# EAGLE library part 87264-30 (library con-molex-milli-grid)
RECEPTACAL
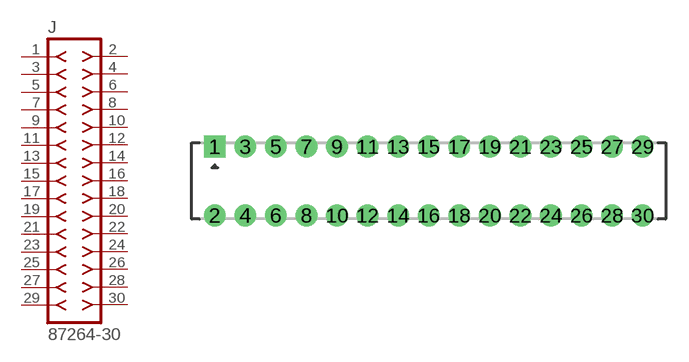
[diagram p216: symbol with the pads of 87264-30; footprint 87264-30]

Designator prefix J

## 87264-30  [87264-30]
1  1  pas
2  2  pas
3  3  pas
4  4  pas
5  5  pas
6  6  pas
7  7  pas
8  8  pas
9  9  pas
10  10  pas
11  11  pas
12  12  pas
13  13  pas
14  14  pas
15  15  pas
16  16  pas
17  17  pas
18  18  pas
19  19  pas
20  20  pas
21  21  pas
22  22  pas
23  23  pas
24  24  pas
25  25  pas
26  26  pas
27  27  pas
28  28  pas
29  29  pas
30  30  pas

## Footprint 87264-30 (pad centres in mm)
RECEPTACAL Dual Row, Side Entry
drill 0.914 square: 1 -14,2.25
drill 0.914: 2 -14,-2.25; 3 -12,2.25; 4 -12,-2.25; 5 -10,2.25; 6 -10,-2.25; 7 -8,2.25; 8 -8,-2.25; 9 -6,2.25; 10 -6,-2.25; 11 -4,2.25; 12 -4,-2.25; 13 -2,2.25; 14 -2,-2.25; 15 0,2.25; 16 0,-2.25; 17 2,2.25; 18 2,-2.25; 19 4,2.25; 20 4,-2.25; 21 6,2.25; 22 6,-2.25; 23 8,2.25; 24 8,-2.25; 25 10,2.25; 26 10,-2.25; 27 12,2.25; 28 12,-2.25; 29 14,2.25; 30 14,-2.25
